[IBIS Ver]   2.1
[File Name]   sprm018.ibs
[File Rev]   0.1
[Date]   February 9, 2001
[Source]   IBIS Model Generated from PACED
[Disclaimer]   Please be aware that in the absence of a written agreement
|   Texas Instruments(TI) assumes no liability for:
|   (1) The accuracy of the IBIS models provided to your company
|   (2) The proper functioning of these Models in your design
|   or for any resulting applications; or
|   (3)Infringement of patents, copyrights or intellectual
|   property rights resulting from your use of these models.
|   TI provides IBIS Models as a service to our customers and
|   therefore reserves the right to limit distribution of the
|   Models.
[Copyright]   Property of Texas Instruments Incorporated.
|   Unauthorized reproduction and/or distribution is strictly.
|   prohibited.
|   This product is protected under copyright law and trade
|   secret law as an unpublished work.
|   Created 1999,(C) Copyright 1999-2000,
|   Texas Instruments Incorporated., All Rights Reserved.
|   These commodities are under the U.S.
|   Government distribution license control. As such,they
|   are not to be re-exported without the prior approval of
|   the U.S.Department of Commerce.
[Component]   c6201_GJC
[Manufacturer]   Texas Instruments
[Package]
| Variable   Typ   Min   Max
R_pkg   0.237   0.1037   0.3935
L_pkg   6.331e-09   2.76e-09   1.05e-08
C_pkg   1.372e-12   6.626e-13   2.207e-12
[Pin]   signal_name  model_name  R_pin   L_pin   C_pin
C10   CLKIN   UIT293   0.2001   5.32E-09   1.15E-12
AF22   CLKOUT1   UOT212   0.2712   7.23E-09   1.52E-12
AF20   CLKOUT2   UOT212   0.2547   6.81E-09   1.43E-12
C6   CLKMODE1   UIT293   0.3935   1.05E-08   2.21E-12
C5   CLKMODE0   UIT293   0.2472   6.60E-09   1.39E-12
A9   PLLFREQ3   UIT293   0.2637   7.01E-09   1.50E-12
D11   PLLFREQ2   UIT293   0.1648   4.38E-09   9.53E-13
B10   PLLFREQ1   UIT293   0.201   5.34E-09   1.17E-12
L3   TMS   UIT293   0.1711   4.54E-09   9.99E-13
W2   TDO   UOT212   0.243   6.48E-09   1.40E-12
R4   TDI   UIT293   0.2134   5.72E-09   1.29E-12
R3   TCK   UIT293   0.1648   4.38E-09   9.68E-13
T1   TRST   UIT293   0.1924   5.15E-09   1.15E-12
Y1   EMU1   UIT285_UOT212   0.2841   7.57E-09   1.62E-12
W3   EMU0   UIT285_UOT212   0.2151   5.73E-09   1.25E-12
K2   RESET   UIT293   0.2033   5.41E-09   1.19E-12
L2   NMI   UIT293   0.2165   5.75E-09   1.28E-12
U3   EXT_INT7   UIT293   0.2031   5.41E-09   1.19E-12
V2   EXT_INT6   UIT293   0.2365   6.30E-09   1.39E-12
W1   EXT_INT5   UIT293   0.2732   7.29E-09   1.58E-12
U4   EXT_INT4   UIT293   0.1752   4.67E-09   1.02E-12
Y2   IACK   UOT212   0.2509   6.70E-09   1.44E-12
AA1   INUM3   UOT212   0.2727   7.27E-09   1.55E-12
W4   INUM2   UOT212   0.1877   5.00E-09   1.07E-12
AA2   INUM1   UOT212   0.2055   5.49E-09   1.17E-12
AB1   INUM0   UOT212   0.2872   7.73E-09   1.67E-12
H3   LENDIAN   UIT293   0.2208   5.88E-09   1.26E-12
D3   PD   UOT212   0.2484   6.64E-09   1.40E-12
H26   HINT   UOT212   0.262   7.10E-09   1.55E-12
F23   HCNTL1   UIT293   0.2031   5.42E-09   1.16E-12
D25   HCNTL0   UIT293   0.2678   7.19E-09   1.53E-12
C26   HHWIL   UIT293   0.2973   8.07E-09   1.74E-12
E23   HBE1   UIT293   0.2067   5.51E-09   1.17E-12
D24   HBE0   UIT293   0.2345   6.25E-09   1.33E-12
C23   HRW   UIT293   0.2963   7.89E-09   1.67E-12
B13   HD15   UIT285_UOT212   0.1986   5.29E-09   1.34E-12
B14   HD14   UIT285_UOT212   0.2007   5.40E-09   1.37E-12
C14   HD13   UIT285_UOT212   0.176   4.72E-09   1.07E-12
B15   HD12   UIT285_UOT212   0.2161   5.75E-09   1.24E-12
D15   HD11   UIT285_UOT212   0.1627   4.32E-09   9.56E-13
B16   HD10   UIT285_UOT212   0.2228   5.92E-09   1.30E-12
A17   HD9   UIT285_UOT212   0.2592   6.91E-09   1.51E-12
B17   HD8   UIT285_UOT212   0.2298   6.11E-09   1.33E-12
D16   HD7   UIT285_UOT212   0.1711   4.54E-09   9.94E-13
B18   HD6   UIT285_UOT212   0.2356   6.30E-09   1.38E-12
A19   HD5   UIT285_UOT212   0.2637   7.04E-09   1.53E-12
C18   HD4   UIT285_UOT212   0.2098   5.60E-09   1.22E-12
B19   HD3   UIT285_UOT212   0.2437   6.48E-09   1.40E-12
C19   HD2   UIT285_UOT212   0.2146   5.71E-09   1.23E-12
B20   HD1   UIT285_UOT212   0.2554   6.80E-09   1.45E-12
B21   HD0   UIT285_UOT212   0.2693   7.21E-09   1.54E-12
C22   HAS   UIT293   0.2787   7.47E-09   1.60E-12
B23   HCS   UIT293   0.2309   6.17E-09   1.31E-12
D22   HDS1   UIT293   0.2602   6.94E-09   1.47E-12
A24   HDS2   UIT293   0.3272   8.73E-09   1.85E-12
J24   HRDY   UOT212   0.2091   5.57E-09   1.21E-12
D8   BOOTMODE4   UIT293   0.1892   5.04E-09   1.08E-12
B4   BOOTMODE3   UIT293   0.2809   7.50E-09   1.58E-12
A3   BOOTMODE2   UIT293   0.3155   8.42E-09   1.77E-12
D5   BOOTMODE1   UIT293   0.2171   5.81E-09   1.22E-12
C4   BOOTMODE0   UIT293   0.2563   6.83E-09   1.43E-12
AE22   CE3   UOT212   0.2688   7.16E-09   1.52E-12
AD26   CE2   UOT212   0.3075   8.22E-09   1.73E-12
AB24   CE1   UOT212   0.2378   6.35E-09   1.35E-12
AC26   CE0   UOT212   0.2894   7.72E-09   1.63E-12
AB25   BE3   UOT212   0.2611   6.97E-09   1.48E-12
AA24   BE2   UOT212   0.2285   6.10E-09   1.30E-12
Y23   BE1   UOT212   0.2231   5.95E-09   1.27E-12
AA26   BE0   UOT212   0.2826   7.64E-09   1.66E-12
J26   EA21   UOT212   0.2554   6.90E-09   1.53E-12
K25   EA20   UOT212   0.2283   6.08E-09   1.33E-12
L24   EA19   UOT212   0.1924   5.12E-09   1.14E-12
K26   EA18   UOT212   0.2631   7.00E-09   1.55E-12
M26   EA17   UOT212   0.2347   6.25E-09   1.44E-12
M25   EA16   UOT212   0.22   5.84E-09   1.31E-12
P25   EA15   UOT212   0.1037   2.76E-09   7.10E-13
P24   EA14   UOT212   0.1876   5.01E-09   1.13E-12
R25   EA13   UOT212   0.1737   4.63E-09   1.04E-12
T26   EA12   UOT212   0.2687   7.26E-09   1.58E-12
R23   EA11   UOT212   0.1929   5.13E-09   1.12E-12
U26   EA10   UOT212   0.2267   6.13E-09   1.35E-12
U25   EA9   UOT212   0.2225   5.92E-09   1.29E-12
T23   EA8   UOT212   0.2125   5.66E-09   1.23E-12
V26   EA7   UOT212   0.2263   6.14E-09   1.36E-12
V25   EA6   UOT212   0.2306   6.16E-09   1.34E-12
W26   EA5   UOT212   0.2612   7.07E-09   1.55E-12
V24   EA4   UOT212   0.2454   6.55E-09   1.43E-12
W25   EA3   UOT212   0.2382   6.34E-09   1.37E-12
Y26   EA2   UOT212   0.2683   7.27E-09   1.59E-12
AB2   ED31   UIT285_UOT212   0.2885   7.78E-09   1.70E-12
AC1   ED30   UIT285_UOT212   0.3065   8.18E-09   1.74E-12
AA4   ED29   UIT285_UOT212   0.2721   7.34E-09   1.58E-12
AD1   ED28   UIT285_UOT212   0.3196   8.53E-09   1.81E-12
AC3   ED27   UIT285_UOT212   0.2503   6.67E-09   1.44E-12
AD4   ED26   UIT285_UOT212   0.2564   6.88E-09   1.49E-12
AF3   ED25   UIT285_UOT212   0.3152   8.49E-09   1.82E-12
AE4   ED24   UIT285_UOT212   0.2829   7.60E-09   1.62E-12
AD5   ED23   UIT285_UOT212   0.2503   6.73E-09   1.44E-12
AF4   ED22   UIT285_UOT212   0.3038   8.19E-09   1.75E-12
AE5   ED21   UIT285_UOT212   0.2763   7.42E-09   1.59E-12
AD6   ED20   UIT285_UOT212   0.2416   6.50E-09   1.39E-12
AE6   ED19   UIT285_UOT212   0.2605   7.01E-09   1.50E-12
AD7   ED18   UIT285_UOT212   0.2315   6.19E-09   1.32E-12
AC8   ED17   UIT285_UOT212   0.1962   5.24E-09   1.13E-12
AF7   ED16   UIT285_UOT212   0.2719   7.25E-09   1.55E-12
AD9   ED15   UIT285_UOT212   0.209   5.58E-09   1.20E-12
AD10   ED14   UIT285_UOT212   0.2   5.34E-09   1.16E-12
AF9   ED13   UIT285_UOT212   0.2596   6.95E-09   1.50E-12
AC11   ED12   UIT285_UOT212   0.1693   4.51E-09   9.98E-13
AE10   ED11   UIT285_UOT212   0.2355   6.29E-09   1.39E-12
AE11   ED10   UIT285_UOT212   0.2152   5.74E-09   1.31E-12
AF11   ED9   UIT285_UOT212   0.244   6.53E-09   1.55E-12
AE14   ED8   UIT285_UOT212   0.2116   5.63E-09   1.36E-12
AF15   ED7   UIT285_UOT212   0.2404   6.39E-09   1.44E-12
AE15   ED6   UIT285_UOT212   0.2186   5.82E-09   1.27E-12
AF16   ED5   UIT285_UOT212   0.2512   6.69E-09   1.44E-12
AC15   ED4   UIT285_UOT212   0.1679   4.47E-09   9.67E-13
AE17   ED3   UIT285_UOT212   0.2405   6.41E-09   1.38E-12
AF18   ED2   UIT285_UOT212   0.2495   6.66E-09   1.44E-12
AF19   ED1   UIT285_UOT212   0.2538   6.77E-09   1.46E-12
AC17   ED0   UIT285_UOT212   0.1811   4.82E-09   1.03E-12
Y24   ARE   UOT212   0.2224   5.93E-09   1.28E-12
AC24   AOE   UOT212   0.2481   6.62E-09   1.41E-12
AD23   AWE   UOT212   0.2593   6.90E-09   1.46E-12
W23   ARDY   UIT293   0.1862   4.96E-09   1.07E-12
AC20   SSADS   UOT212   0.203   5.41E-09   1.15E-12
AF21   SSOE   UOT212   0.2695   7.19E-09   1.51E-12
AD19   SSWE   UOT212   0.2204   5.88E-09   1.25E-12
AD17   SSCLK   UOT212   0.2073   5.52E-09   1.20E-12
AD21   SDA10   UOT212   0.237   6.32E-09   1.34E-12
AF24   SDRAS   UOT212   0.2958   7.92E-09   1.67E-12
AD22   SDCAS   UOT212   0.2483   6.62E-09   1.41E-12
AF23   SDWE   UOT212   0.2884   7.69E-09   1.64E-12
AE20   SDCLK   UOT212   0.2486   6.63E-09   1.40E-12
AA25   HOLD   UIT293   0.2285   6.09E-09   1.30E-12
A7   HOLDA   UIT293_UOT212   0.282   7.51E-09   1.60E-12
H24   TOUT1   UOT212   0.2131   5.70E-09   1.24E-12
K24   TINP1   UIT293   0.1982   5.28E-09   1.16E-12
M4   TOUT0   UOT212   0.2455   6.52E-09   1.46E-12
K4   TINP0   UIT293   0.237   6.30E-09   1.37E-12
E25   CLKS1   UIT293   0.2613   7.02E-09   1.51E-12
H23   CLKR1   UIT285_UOT212   0.1911   5.10E-09   1.10E-12
F26   CLKX1   UIT285_UOT212   0.28   7.55E-09   1.63E-12
D26   DR1   UIT293   0.2922   7.94E-09   1.72E-12
G23   DX1   UOT212   0.1978   5.26E-09   1.13E-12
E26   FSR1   UIT285_UOT212   0.2861   7.78E-09   1.69E-12
F25   FSX1   UIT285_UOT212   0.2558   6.85E-09   1.48E-12
L4   CLKS0   UIT293   0.2225   5.92E-09   1.30E-12
M2   CLKR0   UIT285_UOT212   0.1626   4.33E-09   1.05E-12
L1   CLKX0   UIT285_UOT212   0.22   5.84E-09   1.31E-12
J1   DR0   UIT293   0.1775   4.71E-09   1.03E-12
R1   DX0   UIT285_UOT212   0.1109   2.95E-09   6.63E-13
P4   FSR0   UIT285_UOT212   0.1804   4.79E-09   1.08E-12
P3   FSX0   UIT285_UOT212   0.2509   6.69E-09   1.53E-12
| End of package information
[Component]   UIT293
[Manufacturer]   Texas Instruments
[Package]
|   typ   min   max
R_pkg   0   0   0
L_pkg   0   0   0
C_pkg   0   0   0
[Pin]   signal_name   model_name   R_pin   L_pin   C_pin
   1   A   UIT293   0   0   0
[Component]   UIT285_UOT212
[Manufacturer]   Texas Instruments
[Package]
|   typ   min   max
R_pkg   0   0   0
L_pkg   0   0   0
C_pkg   0   0   0
[Pin]   signal_name   model_name   R_pin   L_pin   C_pin
   1   Y   UIT285_UOT212   0   0   0
[Component]   UIT286
[Manufacturer]   Texas Instruments
[Package]
|   typ   min   max
R_pkg   0   0   0
L_pkg   0   0   0
C_pkg   0   0   0
[Pin]   signal_name   model_name   R_pin   L_pin   C_pin
   1   Y   UIT286   0   0   0
[Component]   UIT293_UOT212
[Manufacturer]   Texas Instruments
[Package]
|   typ   min   max
R_pkg   0   0   0
L_pkg   0   0   0
C_pkg   0   0   0
[Pin]   signal_name   model_name   R_pin   L_pin   C_pin
   1   Y   UIT293_UOT212   0   0   0
[Component]   UOT212
[Manufacturer]   Texas Instruments
[Package]
|   typ   min   max
R_pkg   0   0   0
L_pkg   0   0   0
C_pkg   0   0   0
[Pin]   signal_name   model_name   R_pin   L_pin   C_pin
   1   Y   UOT212   0   0   0
[Component]   UIT293_UPT219
[Manufacturer]   Texas Instruments
[Package]
|   typ   min   max
R_pkg   0   0   0
L_pkg   0   0   0
C_pkg   0   0   0
[Pin]   signal_name   model_name   R_pin   L_pin   C_pin
   1   A   UIT293_UPT219   0   0   0
| Models and submodels in the file (6): UIT293 (Input), UIT285_UOT212 (I/O), UIT286 (Input), UIT293_UOT212 (I/O), UOT212 (3-state), UIT293_UPT219 (Input)
